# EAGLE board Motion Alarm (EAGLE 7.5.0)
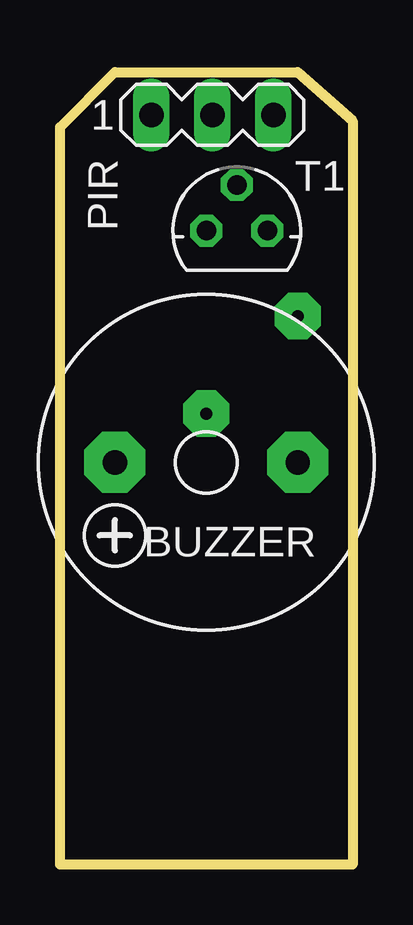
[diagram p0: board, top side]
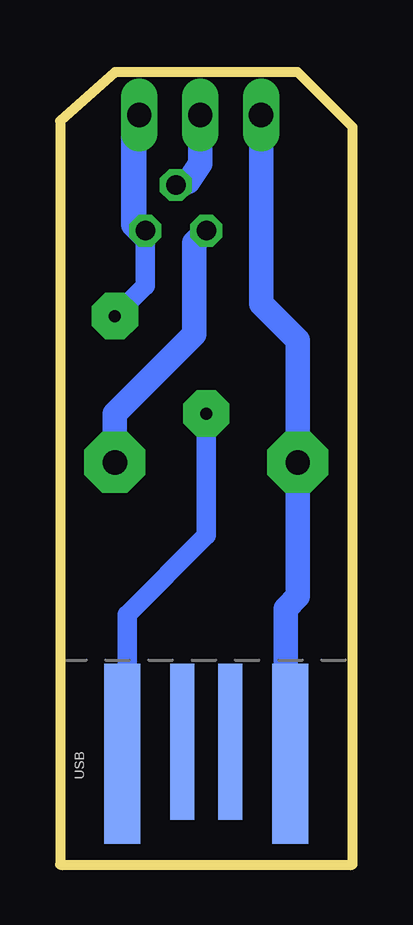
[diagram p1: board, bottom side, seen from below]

Size 12.19 x 33.02 mm. Coordinates in mm from the lower left corner, seen from the top.
Outline: 12.19,30.99 12.19,0 0,0 0,30.73 2.29,33.02 9.91,33.02 12.19,30.99
Copper layers (1*16): Top 0.035mm / dielectric 1.5mm / Bottom 0.035mm
Design rules "default": minimum track width 10mil, minimum drill 24mil, track to track 8mil, track to pad 8mil, pad to pad 8mil, via to via 8mil, smd to smd 8mil, copper to edge 40mil, drill to drill 8mil, minimum pad ring 10mil, minimum via ring 8mil, stop-mask expansion 4mil, vias tented up to drill 0mil, thermal gap 10mil

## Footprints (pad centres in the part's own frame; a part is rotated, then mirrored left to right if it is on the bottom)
F/CM12P = drill 1.016 pad 2.54 octagon: + 3.81,0; - -3.81,0
MA03-1 = drill 1.016 long: 1 -2.54,0; 2 0,0; 3 2.54,0
78LXX = drill 0.813 octagon: GND 0,1.905; IN 1.27,0; OUT -1.27,0
USB-A-PCB = smd 7.5 x 1.5: 5V -0.2,-3.5; GND -0.2,3.5 | smd 6.5 x 1: USB_M 0.3,-1; USB_P 0.3,1

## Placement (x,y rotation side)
BUZZER  [F/CM12P]  6.1,16.76 180 top
PIR  [MA03-1]  6.35,31.24 0 top
T1  [78LXX]  7.37,26.42 0 top
USB  [USB-A-PCB]  6.1,4.83 90 bottom

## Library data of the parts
BUZZER = buzzer
PIR = con-lstb
T1 = v-reg
USB = SparkFun-Connectors

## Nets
S$1: BUZZER.+ PIR.1
S$2: PIR.2
S$3: BUZZER.- T1.OUT
S$4: PIR.3 T1.IN

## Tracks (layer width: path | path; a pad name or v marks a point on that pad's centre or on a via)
S$1
  Bottom 1.016: PIR.1 3.81,23.37 2.29,21.84 BUZZER.+ 2.29,11.18 2.79,10.67 2.79,4.83
S$2
  Bottom 1.016: 7.37,28.19 6.86,28.45 6.35,29.21 PIR.2
S$3
  Bottom 1.016: T1.OUT 6.6,25.91 6.6,22.1 9.91,18.8 BUZZER.-
S$4  (via drill 0.5 pad 1.93)
  Bottom 0.61: PIR.3 8.89,26.67 T1.IN
  Bottom 0.813: T1.IN 8.64,24.13 v9.91,22.86
S$5
  Bottom 0.61: 9.91,6.35 9.4,5.84
S$6
  Bottom 1.016: 8.64,26.16 9.14,26.67 9.14,31.24
S$7  (via drill 0.5 pad 1.93)
  Bottom 0.813: v6.1,18.8 6.1,13.72 9.4,10.41 9.4,5.59 9.65,5.33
